// TwinCAT 3 PLC project mongodb
// ProgramVersion: 3.1.4023.0
// libraries:
//   Tc2_Standard, * (Beckhoff Automation GmbH)
//   Tc2_System, * (Beckhoff Automation GmbH)
//   Tc3_Database, * (Beckhoff Automation GmbH)
//   Tc3_Module, * (Beckhoff Automation GmbH)
// project tree:
//   DUTs/ eMyDbState.TcDUT
//   / PlcTask.TcTTO
//   POUs/ MongoDB.TcPOU
// real-time tasks:
//   TASK PlcTask: cycle T#10ms, priority 20, ADS port 350
//   TASK PlcTask1: cycle T#10ms, priority 21, ADS port 351

CONFIGURATION mongodb
    RESOURCE PLC ON TwinCAT3
        TASK PlcTask(INTERVAL := T#10ms, PRIORITY := 20);
        PROGRAM MongoDB WITH PlcTask : MongoDB;
    END_RESOURCE
END_CONFIGURATION

// ---- DUTs/eMyDbState.TcDUT
{attribute 'qualified_only'}
{attribute 'strict'}
TYPE eMyDbState :
(
	aggregation := 0,
	error := 10,
	idle := 20,
	readstruct := 30,
	validationissues := 40,
	validationremaining := 50,
	write := 60,
	createcollection := 70,
	dropcollection := 80,
	updateone := 90,
	updatemany := 100,
	writemany := 110,
	delete := 120,
	deletemany := 130
);
END_TYPE

// ---- POUs/MongoDB.TcPOU
PROGRAM MongoDB
VAR
	// 数据库功能块
	fbNoSQLQueryBuilder_DocumentDB: FB_NoSQLQueryBuilder_DocumentDB;
	// 数据库请求命令
	fbNoSqlQuery : FB_NoSQLQueryEvt(sNetID := '', tTimeout := T#5S);
	// 数据库返回值
	fbNoSqlResult : FB_NoSQLResultEvt(sNetID := '', tTimeout := T#5S);
	// 
	fbNoSqlValidation : FB_NoSQLValidationEvt(sNetID := '', tTimeout := TIME#15S0MS);
	// case步变量
	eState : eMyDbState := eMyDbState.idle;
	// Eventlog信息
	InfoResult: Tc3_Database.I_TcMessage;
	
	// 数据库信息
	// 数据库ID
	myDBID : UDINT := 1;
	// 数据集名称
	myDataset : STRING := 'twincat';
	// 测试用数据集名称
	testDataset : STRING := 'twincat2';
	
	// json字符串
	// 请求字符串
	queryDocument : STRING(1000) := '{demostr : "demodata"}';
	// 数据聚合
	sPipeStages: STRING(1000) := '{$$match :{Name : "Some Name Value"}}';
	// 写入数据
	writeDocument : STRING(1000) := '{"demostr" : "demodata", "demobool" : true, "demonum" : 2.3}';
	// 批量插入数据
	writeManyDocument: STRING(1000) := '[{"demostr" : "demodata", "demobool" : true, "demonum" : 2.3}, 
										 {"demostr" : "demodata", "demobool" : true, "demonum" : 2.4}, 
										 {"demostr" : "demodata", "demobool" : true, "demonum" : 2.5}]';
	// 读取数据（20条）
	dataDocument : ARRAY[1..20] OF STRING(1000);
	// 升级数据
	updatequeryDocument : STRING(1000) := '{"demobool" : true}';
	updateDocument : STRING(1000) := '{$$set : {"demobool" : false}}';
	// 删除数据
	deleteDocument : STRING(1000) := '{"demonum" : 2.3}';
	
	// 
	aIssues : ARRAY[0..99] OF STRING(512);
	// 
    aRemaining : ARRAY [0..9] OF STRING(1000);
	
	// 命令
	// 数据聚合
	AggregateQueryOptions : Tc3_Database.T_QueryOptionDocumentDB_Aggregate;
	// 数据删除
	DeleteQueryOptions : Tc3_Database.T_QueryOptionDocumentDB_Delete;
	// 数据插入
	InsertQueryOptions : Tc3_Database.T_QueryOptionDocumentDB_Insert;
	// 数据查询
	FindQueryOptions : Tc3_Database.T_QueryOptionDocumentDB_Find;
	// 数据更新
	UpdateQueryOptions : Tc3_Database.T_QueryOptionDocumentDB_Update;
END_VAR

CASE eState OF
	
	eMyDbState.aggregation:
		// 数据聚合
		aggregation();

	eMyDbState.error:
		// 出现错误

	eMyDbState.idle:
		// 

	eMyDbState.readstruct:
		// 从数据库读取数据
		readdata();
	
	eMyDbState.validationissues:
		// 
		getvalidationissue();
	
	eMyDbState.validationremaining:
		// 
		getvalidationremaining();
		
	eMyDbState.write:
		// 向数据库写入单个数据
		writedata();
		
	eMyDbState.createcollection:
		// 创建数据集
		createcollection();
		
	eMyDbState.dropcollection:
		// 删除数据集
		dropcollection();
		
	eMyDbState.updateone:
		// 更新数据
		updateone();
		
	eMyDbState.updatemany:
		// 批量更新
		updatemany();
		
	eMyDbState.writemany:
		// 批量写入
		writemany();
		
	eMyDbState.delete:
		// 删除数据
		deletedata();
		
	eMyDbState.deletemany:
		// 批量删除数据
		deletemanydata();
	
END_CASE

ACTION aggregation:
(*
MongoDB 中聚合(aggregate)主要用于处理数据(诸如统计平均值，求和等)，并返回计算后的数据结果。
有点类似 SQL 语句中的 count。
MongoDB中聚合的方法使用aggregate()。
命令参考：
db.COLLECTION_NAME.aggregate(AGGREGATE_OPERATION)
*)

// 请求字符串
// AGGREGATE_OPTION，可以使用聚合表达式或者是管道命令进行操作
AggregateQueryOptions.pPipeStages := ADR(sPipeStages);
AggregateQueryOptions.cbPipeStages := SIZEOF(sPipeStages);

// 请求命令
// 使用aggregation命令进行插入
fbNoSQLQueryBuilder_DocumentDB.eQueryType := E_DocumentDbQueryType.Aggregation;
// 数据集名称，默认是twincat
fbNoSQLQueryBuilder_DocumentDB.sCollectionName := myDataset;
// 请求字符串的地址以及长度
fbNoSQLQueryBuilder_DocumentDB.pQueryOptions := ADR(AggregateQueryOptions);
fbNoSQLQueryBuilder_DocumentDB.cbQueryOptions := SIZEOF(AggregateQueryOptions);

// 发送请求命令
// 请求返回至fbnosqlresult功能块
IF fbNoSqlQuery.ExecuteDataReturn(hDBID:= myDBID, iNoSQLQueryBuilder:= fbNoSQLQueryBuilder_DocumentDB, pNoSQLResult:= ADR(fbNoSqlResult)) THEN
	// 发生报错则记录系统信息
	IF fbNoSqlQuery.bError THEN
		InfoResult := fbNoSqlQuery.ipTcResult;
		eState:= eMyDbState.Error;
	ELSE
		// 结果转存到datadocument数组当中，返回值是json字符串
		IF fbNoSqlResult.ReadAsString(nStartIndex:= 0, nRecordCount:= 20, pData:= ADR(dataDocument), cbData:= SIZEOF(dataDocument), 
			MaxDocumentSize:= SIZEOF(dataDocument[1]), bDataRelease:= TRUE) THEN
			IF fbNoSqlResult.bError THEN
				InfoResult := fbNoSqlResult.ipTcResult;
				eState := eMyDbState.error;
			ELSE
				eState:= eMyDbState.Idle; 
			END_IF
		END_IF
	END_IF
END_IF
END_ACTION

ACTION createcollection:
(*
MongoDB 中使用 **createCollection()** 方法来创建集合
命令参考：
db.createCollection(name, options)
*)

// 请求命令
fbNoSQLQueryBuilder_DocumentDB.eQueryType := E_DocumentDbQueryType.CreateCollection;
// 创建的数据集名称为testDataset字符串的内容
fbNoSQLQueryBuilder_DocumentDB.sCollectionName := testDataset;

// 发送请求命令
IF fbNoSQLQuery.Execute(myDBID, fbNoSQLQueryBuilder_DocumentDB) THEN
	IF fbNoSQLQuery.bError THEN
		InfoResult := fbNoSQLQuery.ipTcResult;
		eState:= eMyDbState.Error;
	ELSE
		eState:= eMyDbState.Idle; 
	END_IF
END_IF
END_ACTION

ACTION deletedata:
(*
MongoDB remove()函数是用来移除集合中的数据。
命令参考：
db.collection.remove(
   <query>,
   <justOne>
)
*)

// 请求字符串
// <query> : 删除命令的查询条件
DeleteQueryOptions.pFilter:= ADR(deleteDocument);
DeleteQueryOptions.cbFilter:= SIZEOF(deleteDocument); 

// 请求命令
// 使用delete命令进行删除
fbNoSQLQueryBuilder_DocumentDB.eQueryType := Tc3_Database.E_DocumentDbQueryType.Delete;
// 数据集名称，默认是twincat
fbNoSQLQueryBuilder_DocumentDB.sCollectionName := myDataset;
// 请求字符串的地址以及长度
fbNoSQLQueryBuilder_DocumentDB.pQueryOptions := ADR(DeleteQueryOptions);
fbNoSQLQueryBuilder_DocumentDB.cbQueryOptions := SIZEOF(DeleteQueryOptions);

// 发送请求命令
IF fbNoSQLQuery.Execute(myDBID, fbNoSQLQueryBuilder_DocumentDB) THEN
	// 发生报错则记录系统信息
	IF fbNoSQLQuery.bError THEN
		InfoResult := fbNoSQLQuery.ipTcResult;
		eState:= eMyDbState.Error;
	ELSE
		eState:= eMyDbState.Idle; 
	END_IF
END_IF
END_ACTION

ACTION deletemanydata:
(*
说明参考deletedata
*)

// 请求字符串
DeleteQueryOptions.pFilter:= ADR(deleteDocument);
DeleteQueryOptions.cbFilter:= SIZEOF(deleteDocument); 

// 请求命令
fbNoSQLQueryBuilder_DocumentDB.eQueryType := Tc3_Database.E_DocumentDbQueryType.DeleteMany;
fbNoSQLQueryBuilder_DocumentDB.sCollectionName := myDataset;
fbNoSQLQueryBuilder_DocumentDB.pQueryOptions := ADR(DeleteQueryOptions);
fbNoSQLQueryBuilder_DocumentDB.cbQueryOptions := SIZEOF(DeleteQueryOptions);

// 发送请求命令
IF fbNoSQLQuery.Execute(myDBID, fbNoSQLQueryBuilder_DocumentDB) THEN
	IF fbNoSQLQuery.bError THEN
		InfoResult := fbNoSQLQuery.ipTcResult;
		eState:= eMyDbState.Error;
	ELSE
		eState:= eMyDbState.Idle; 
	END_IF
END_IF
END_ACTION

ACTION dropcollection:
(*
参考方法createcollection
*)

// 请求命令
fbNoSQLQueryBuilder_DocumentDB.eQueryType := E_DocumentDbQueryType.DropCollection;
fbNoSQLQueryBuilder_DocumentDB.sCollectionName := testDataset;

// 发送请求命令
IF fbNoSQLQuery.Execute(myDBID, fbNoSQLQueryBuilder_DocumentDB) THEN
	IF fbNoSQLQuery.bError THEN
		InfoResult := fbNoSQLQuery.ipTcResult;
		eState:= eMyDbState.Error;
	ELSE
		eState:= eMyDbState.Idle; 
	END_IF
END_IF
END_ACTION

ACTION getvalidationissue:
IF fbNoSqlValidation.GetIssues(pData:= ADR(aIssues), cbData:= SIZEOF(aIssues), bDataRelease:= FALSE) THEN
	IF fbNoSqlValidation.bError THEN
		InfoResult := fbNoSqlValidation.ipTcResult;
		eState := eMyDbState.error;
	ELSE
		eState := eMyDbState.idle;
	END_IF
END_IF
END_ACTION

ACTION getvalidationremaining:
IF fbNoSqlValidation.GetRemainingData(pData:= ADR(aRemaining), cbData:= SIZEOF(aRemaining), cbDocument:= SIZEOF(aRemaining[1]), bDataRelease:= FALSE) THEN
	IF fbNoSqlValidation.bError THEN
		InfoResult := fbNoSqlValidation.ipTcResult;
		eState := eMyDbState.error;
	ELSE
		eState := eMyDbState.idle;
	END_IF
END_IF
END_ACTION

ACTION readdata:
(*
mongodb使用find函数查询数据
命令参考：
db.collection.find(<query>, projection)
*)

// 请求字符串
// find命令的请求条件
FindQueryOptions.pFilter:= ADR(queryDocument);
FindQueryOptions.cbFilter:= SIZEOF(queryDocument); 

// 请求命令
// 使用find命令进行查找
fbNoSQLQueryBuilder_DocumentDB.eQueryType := Tc3_Database.E_DocumentDbQueryType.Find;
// 数据集名称，默认是twincat
fbNoSQLQueryBuilder_DocumentDB.sCollectionName := myDataset;
// 请求字符串的地址以及长度
fbNoSQLQueryBuilder_DocumentDB.pQueryOptions := ADR(FindQueryOptions);
fbNoSQLQueryBuilder_DocumentDB.cbQueryOptions := SIZEOF(FindQueryOptions);

// 发送请求命令
// 请求返回至fbnosqlresult功能块
IF fbNoSqlQuery.ExecuteDataReturn(hDBID:= myDBID, iNoSQLQueryBuilder:= fbNoSQLQueryBuilder_DocumentDB, pNoSQLResult:= ADR(fbNoSqlResult)) THEN
	// 发生报错则记录系统信息
	IF fbNoSqlQuery.bError THEN
		InfoResult := fbNoSqlQuery.ipTcResult;
		eState:= eMyDbState.Error;
	ELSE
		// 结果转存到datadocument数组当中，读取出来的是json字符串
		IF fbNoSqlResult.ReadAsString(nStartIndex:= 0, nRecordCount:= 20, pData:= ADR(dataDocument), cbData:= SIZEOF(dataDocument), 
			MaxDocumentSize:= SIZEOF(dataDocument[1]), bDataRelease:= TRUE) THEN
			IF fbNoSqlResult.bError THEN
				InfoResult := fbNoSqlResult.ipTcResult;
				eState := eMyDbState.error;
			ELSE
				eState:= eMyDbState.Idle; 
			END_IF
		END_IF
	END_IF
END_IF
END_ACTION

ACTION updatemany:
(*
说明参考updateone
*)

// 请求字符串
UpdateQueryOptions.pFilter := ADR(updatequeryDocument);
UpdateQueryOptions.cbFilter := SIZEOF(updatequeryDocument);
UpdateQueryOptions.pDocuments := ADR(updateDocument);
UpdateQueryOptions.cbDocuments := SIZEOF(updateDocument);

// 请求命令
fbNoSQLQueryBuilder_DocumentDB.eQueryType := E_DocumentDbQueryType.UpdateMany;
fbNoSQLQueryBuilder_DocumentDB.sCollectionName := myDataset;
fbNoSQLQueryBuilder_DocumentDB.pQueryOptions := ADR(UpdateQueryOptions);
fbNoSQLQueryBuilder_DocumentDB.cbQueryOptions := SIZEOF(UpdateQueryOptions);

// 发送请求命令
IF fbNoSQLQuery.Execute(myDBID, fbNoSQLQueryBuilder_DocumentDB) THEN
	IF fbNoSQLQuery.bError THEN
		InfoResult := fbNoSQLQuery.ipTcResult;
		eState:= eMyDbState.Error;
	ELSE
		eState:= eMyDbState.Idle; 
	END_IF
END_IF
END_ACTION

ACTION updateone:
(*
update方法用于更新已存在的文档
命令参考：
db.collection.update(
   <query>,
   <update>,
   {
     upsert: <boolean>,
     multi: <boolean>,
     writeConcern: <document>
   }
)
*)

// 请求字符串
// <query> : update的查询条件，类似sql update查询内where后面的
UpdateQueryOptions.pFilter := ADR(updatequeryDocument);
UpdateQueryOptions.cbFilter := SIZEOF(updatequeryDocument);
// <update> : 更新内容
UpdateQueryOptions.pDocuments := ADR(updateDocument);
UpdateQueryOptions.cbDocuments := SIZEOF(updateDocument);

// 请求命令
// 使用updateone命令进行更新
fbNoSQLQueryBuilder_DocumentDB.eQueryType := E_DocumentDbQueryType.UpdateOne;
// 数据集名称，默认是twincat
fbNoSQLQueryBuilder_DocumentDB.sCollectionName := myDataset;
fbNoSQLQueryBuilder_DocumentDB.sCollectionName := myDataset;
// 请求字符串的地址以及长度
fbNoSQLQueryBuilder_DocumentDB.pQueryOptions := ADR(UpdateQueryOptions);
fbNoSQLQueryBuilder_DocumentDB.cbQueryOptions := SIZEOF(UpdateQueryOptions);

// 发送请求命令
IF fbNoSQLQuery.Execute(myDBID, fbNoSQLQueryBuilder_DocumentDB) THEN
	// 发生报错则记录系统信息
	IF fbNoSQLQuery.bError THEN
		InfoResult := fbNoSQLQuery.ipTcResult;
		eState:= eMyDbState.Error;
	ELSE
		eState:= eMyDbState.Idle; 
	END_IF
END_IF
END_ACTION

ACTION writedata:
(*
MongoDB以BSON的方式进行文件存储，BSON格式是JSON格式的二进制化存储。文件会被存储在集中。
文中的例子表示向库存集合中插入新的文档。如果未指定_id字段，那么数据库将具有ObjectId值的Id字段添加到新文件中。
命令参考：
db.inventory.insertOne(
   { "item" : "canvas",
     "qty" : 100,
     "tags" : ["cotton"],
     "size" : { "h" : 28, "w" : 35.5, "uom" : "cm" }
   }
)
*)

// 请求字符串
InsertQueryOptions.pDocuments:= ADR(writeDocument); 
InsertQueryOptions.cbDocuments:= SIZEOF(writeDocument);

// 请求命令
// 使用insert命令进行插入
fbNoSQLQueryBuilder_DocumentDB.eQueryType := E_DocumentDbQueryType.InsertOne;
// 数据集名称，默认是twincat
fbNoSQLQueryBuilder_DocumentDB.sCollectionName := myDataset;
// 请求字符串的地址以及长度
fbNoSQLQueryBuilder_DocumentDB.pQueryOptions := ADR(InsertQueryOptions);
fbNoSQLQueryBuilder_DocumentDB.cbQueryOptions := SIZEOF(InsertQueryOptions);

// 发送请求命令
IF fbNoSQLQuery.Execute(myDBID, fbNoSQLQueryBuilder_DocumentDB) THEN
	// 发生报错则记录系统信息
	IF fbNoSQLQuery.bError THEN
		InfoResult := fbNoSQLQuery.ipTcResult;
		eState:= eMyDbState.Error;
	ELSE
		eState:= eMyDbState.Idle; 
	END_IF
END_IF
END_ACTION

ACTION writemany:
(*
命令参考：
db.collection.insertMany(
   [ <document 1> , <document 2>, ... ],
   {
      writeConcern: <document>,
      ordered: <boolean>
   }
)
*)

// 请求字符串
InsertQueryOptions.pDocuments:= ADR(writeManyDocument); 
InsertQueryOptions.cbDocuments:= SIZEOF(writeManyDocument);

// 请求命令
// 使用insertmany命令进行插入
fbNoSQLQueryBuilder_DocumentDB.eQueryType := E_DocumentDbQueryType.InsertMany;
// 数据集名称，默认是twincat
fbNoSQLQueryBuilder_DocumentDB.sCollectionName := myDataset;
// 请求字符串的地址以及长度
fbNoSQLQueryBuilder_DocumentDB.pQueryOptions := ADR(InsertQueryOptions);
fbNoSQLQueryBuilder_DocumentDB.cbQueryOptions := SIZEOF(InsertQueryOptions);

// 发送请求命令
IF fbNoSQLQuery.Execute(myDBID, fbNoSQLQueryBuilder_DocumentDB) THEN
	// 发生报错则记录系统信息
	IF fbNoSQLQuery.bError THEN
		InfoResult := fbNoSQLQuery.ipTcResult;
		eState:= eMyDbState.Error;
	ELSE
		eState:= eMyDbState.Idle; 
	END_IF
END_IF
END_ACTION

END_PROGRAM
